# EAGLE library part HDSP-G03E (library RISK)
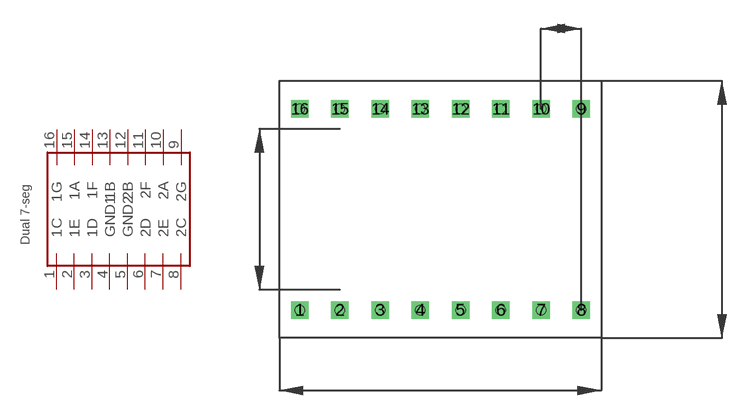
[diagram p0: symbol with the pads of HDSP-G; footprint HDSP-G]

Designator prefix -

## HDSP-G03E  [HDSP-G]
1  1C
2  1E
3  1D
4  GND1
5  GND2
6  2D
7  2E
8  2C
9  2G
10  2A
11  2F
12  2B
13  1B
14  1F
15  1A
16  1G

## Footprint HDSP-G (pad centres in mm)
drill 0.6 square: 1 -8.89,-6.35; 2 -6.35,-6.35; 3 -3.81,-6.35; 4 -1.27,-6.35; 5 1.27,-6.35; 6 3.81,-6.35; 7 6.35,-6.35; 8 8.89,-6.35; 9 8.89,6.35; 10 6.35,6.35; 11 3.81,6.35; 12 1.27,6.35; 13 -1.27,6.35; 14 -3.81,6.35; 15 -6.35,6.35; 16 -8.89,6.35
hole 0.6 at 1.27,-6.35
hole 0.6 at 1.27,-6.35
hole 0.6 at 1.27,-6.35
hole 0.6 at 1.27,-6.35
hole 0.6 at -1.27,-6.35
hole 0.6 at -1.27,-6.35
hole 0.6 at -3.81,-6.35
hole 0.6 at -3.81,-6.35
hole 0.6 at -6.35,-6.35
hole 0.6 at -6.35,-6.35
hole 0.6 at -6.35,-6.35
hole 0.6 at -8.89,-6.35
hole 0.6 at -8.89,-6.35
hole 0.6 at 3.81,-6.35
hole 0.6 at 3.81,-6.35
hole 0.6 at 3.81,-6.35
hole 0.6 at 6.35,-6.35
hole 0.6 at 6.35,-6.35
hole 0.6 at 8.89,-6.35
hole 0.6 at 8.89,-6.35
hole 0.6 at 8.89,-6.35
hole 0.6 at 8.89,6.35
hole 0.6 at 8.89,6.35
hole 0.6 at 6.35,6.35
hole 0.6 at 6.35,6.35
hole 0.6 at 3.81,6.35
hole 0.6 at 3.81,6.35
hole 0.6 at 1.27,6.35
hole 0.6 at 1.27,6.35
hole 0.6 at -1.27,6.35
hole 0.6 at -1.27,6.35
hole 0.6 at -3.81,6.35
hole 0.6 at -3.81,6.35
hole 0.6 at -6.35,6.35
hole 0.6 at -6.35,6.35
hole 0.6 at -6.35,6.35
hole 0.6 at -8.89,6.35
hole 0.6 at -8.89,6.35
